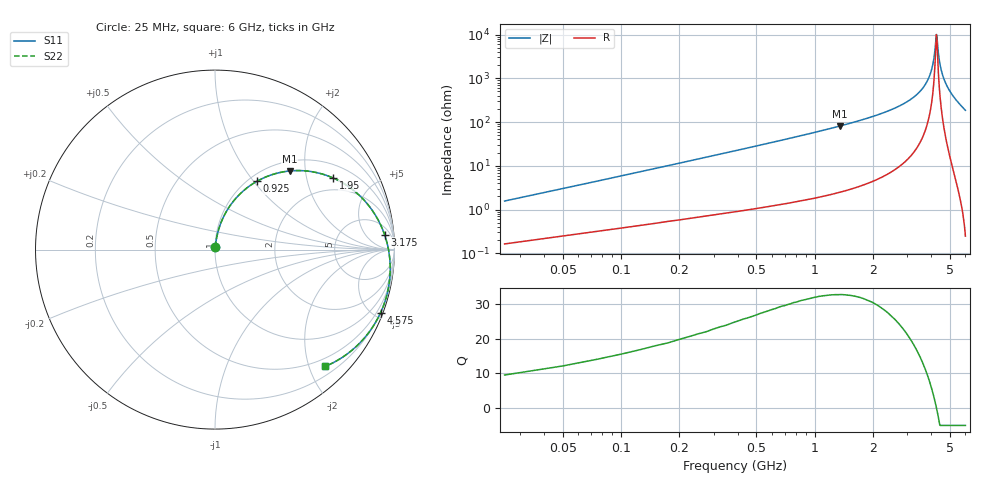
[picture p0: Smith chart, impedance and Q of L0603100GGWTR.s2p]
!	AVX Thin Film Operation
!	Date:	March	2003
!	Description: Accu-L® Series Thin Film SMD RF Inductors
!	Part Number: L0603100GGWTR
!	25MHz-6GHz
!	Serial	Measurements
#	mhz	S	db	R	50
!	S11	S11	S21	S21	S12	S12	S22	S22
!	dB	Phase	dB	Phase	dB	Phase	dB	Phase
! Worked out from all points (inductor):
!   240 points, 25 MHz to 6 GHz, reference 50 ohm
!   read as one part in series: L = 9.44 nH near 50 MHz
!   highest Q = 32.6 at 1.35 GHz (marker M1), where L = 9.59 nH
!   self-resonance near 4.25 GHz
!   S11 on the Smith chart (normalised r, x): 25 MHz: 1.00, +0.03; 925 MHz: 1.09, +1.04; 1.95 GHz: 1.47, +2.89; 3.175 GHz: 10, +17; 4.575 GHz: 0.20, -5.43; 6 GHz: 0.35, -2.28
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25  -36.50 82.7  -0.01 -0.9  -0.01 -0.9  -36.50 82.7
50  -30.82 83.2  -0.03 -1.8  -0.03 -1.8  -30.82 83.2
100  -25.08 82.6  -0.05 -3.5  -0.05 -3.5  -25.08 82.6
250  -17.45 78.6  -0.14 -8.5  -0.14 -8.5  -17.45 78.6
525  -11.36 70.3  -0.42 -17.4  -0.42 -17.4  -11.36 70.3
925  -6.98 58.4  -1.11 -29.6  -1.11 -29.6  -6.98 58.4
1025  -6.24 55.5  -1.33 -32.6  -1.33 -32.6  -6.24 55.5
1350  -4.37 46.5  -2.16 -41.6  -2.16 -41.6  -4.37 46.5
1950  -2.28 31.3  -4.19 -56.7  -4.19 -56.7  -2.28 31.3
2025  -2.09 29.5  -4.49 -58.5  -4.49 -58.5  -2.09 29.5
3025  -0.58 8.0  -9.89 -79.2  -9.89 -79.2  -0.58 8.0
3175  -0.46 5.1  -11.05 -81.9  -11.05 -81.9  -0.46 5.1
3700  -0.18 -4.9  -16.94 -89.9  -16.94 -89.9  -0.18 -4.9
4025  -0.10 -10.9  -24.54 -90.4  -24.54 -90.4  -0.10 -10.9
4150  -0.09 -13.2  -30.91 -82.3  -30.91 -82.3  -0.09 -13.2
4250  -0.08 -15.0  -40.27 -23.1  -40.27 -23.1  -0.08 -15.0
4275  -0.08 -15.4  -39.44 12.1  -39.44 12.1  -0.08 -15.4
4350  -0.09 -16.8  -31.90 52.3  -31.90 52.3  -0.09 -16.8
4400  -0.09 -17.7  -28.56 58.7  -28.56 58.7  -0.09 -17.7
4575  -0.11 -20.8  -21.91 63.6  -21.91 63.6  -0.11 -20.8
5025  -0.25 -28.9  -14.39 59.5  -14.39 59.5  -0.25 -28.9
6000  -0.96 -46.6  -7.48 43.6  -7.48 43.6  -0.96 -46.6
